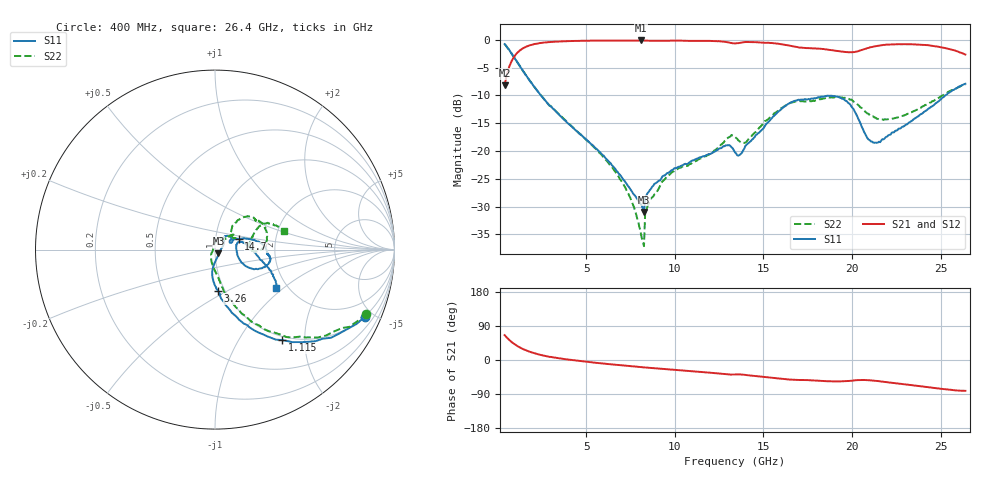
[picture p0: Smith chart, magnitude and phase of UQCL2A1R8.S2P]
! AVX Corporation
! Date:  10/27/06
! Part No:  UQCL2A1R8
! Description:  Ultra Low ESR Microwave capacitors
! Mounting Orientation:  Horizontal
# GHZ S DB R 50
! Freq  |S11|  S11 Ph  |S21|  S21 Ph  |S12|  S12 Ph  |S22|  S22 Ph
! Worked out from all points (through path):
!   401 points, 400 MHz to 26.4 GHz, reference 50 ohm
!   highest |S21| = -0.12 dB at 8.07 GHz (marker M1); lowest = -8.2 dB at 400 MHz (marker M2)
!   group delay of S21, straight-line fit = 10.9 ps
!   lowest |S11| = -31.0 dB at 8.265 GHz (marker M3), VSWR 1.06, Z = 51.9 - j2.14 ohm
!   |S11| at or under -10 dB: 2.447 GHz to 25.27 GHz (22.83 GHz wide, 165 % of centre)
!   |S22| runs from -37.1 to -0.8 dB; largest |S21 - S12| = 0.008
!   S11 on the Smith chart (normalised r, x): 400 MHz: 0.97, -4.44; 1.115 GHz: 0.94, -1.57; 3.26 GHz: 0.93, -0.45; 14.7 GHz: 1.29, +0.15; 26.4 GHz: 1.76, -0.89
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0.4  -0.78 -24.3  -8.19 65.7  -8.19 65.5  -0.76 -23.0
1.115  -4.03 -53.3  -2.33 37.0  -2.36 36.6  -4.03 -50.8
1.96  -7.95 -71.8  -0.87 19.6  -0.87 19.9  -7.97 -66.1
3.26  -12.76 -85.9  -0.34 6.1  -0.35 6.2  -12.72 -78.3
4.755  -17.20 -96.1  -0.19 -3.4  -0.20 -3.4  -17.26 -86.4
7.095  -25.12 -82.8  -0.13 -14.5  -0.13 -14.5  -25.94 -115.9
8.07  -29.49 -55.3  -0.12 -18.6  -0.13 -18.6  -34.49 -141.5
8.265  -30.97 -46.7  -0.15 -19.5  -0.14 -19.4  -37.11 -150.8
8.46  -27.61 17.1  -0.17 -20.2  -0.17 -20.2  -29.94 101.8
9.11  -25.32 30.6  -0.18 -22.7  -0.18 -22.7  -26.68 85.8
9.89  -23.39 42.4  -0.15 -25.5  -0.15 -25.5  -23.70 68.0
12.815  -19.14 39.5  -0.37 -37.3  -0.36 -37.2  -18.21 42.0
13.4  -20.23 22.1  -0.66 -38.1  -0.67 -38.1  -17.48 30.5
13.92  -19.59 32.5  -0.42 -38.9  -0.42 -39.0  -18.54 38.8
14.7  -16.80 23.9  -0.45 -43.2  -0.46 -43.2  -16.12 52.5
16.39  -11.55 6.9  -1.01 -51.2  -1.00 -51.2  -11.59 44.7
17.755  -10.56 -5.0  -1.51 -53.6  -1.51 -53.6  -11.02 34.9
19.64  -10.95 -20.9  -2.20 -56.0  -2.20 -55.9  -10.45 14.4
21.135  -18.30 -3.8  -1.29 -54.2  -1.30 -54.3  -13.77 -1.4
22.11  -17.09 18.2  -0.85 -59.4  -0.85 -59.5  -14.23 9.3
24.515  -11.98 -11.2  -1.07 -73.0  -1.07 -73.1  -11.07 27.6
26.4  -7.91 -31.7  -2.65 -81.4  -2.66 -81.8  -8.03 14.8
